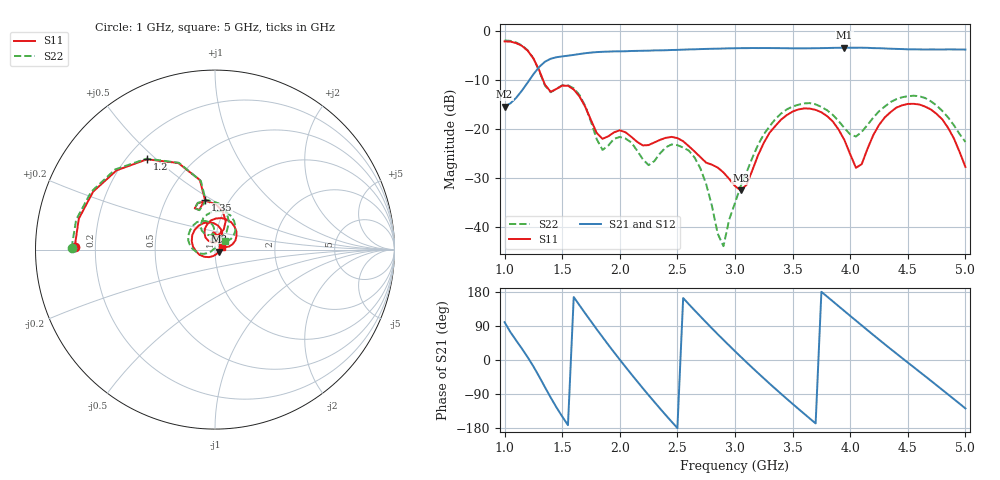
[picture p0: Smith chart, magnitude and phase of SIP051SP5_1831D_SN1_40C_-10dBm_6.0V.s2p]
# GHz  S  dB  R  50
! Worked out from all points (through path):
!   81 points, 1 GHz to 5 GHz, reference 50 ohm
!   highest |S21| = -3.42 dB at 3.95 GHz (marker M1); lowest = -15.5 dB at 1 GHz (marker M2)
!   lowest |S11| = -32.6 dB at 3.05 GHz (marker M3), VSWR 1.05, Z = 52.1 - j1.21 ohm
!   |S11| at or under -10 dB: 1.333 GHz to end of sweep
!   |S22| runs from -44.0 to -1.9 dB; largest |S21 - S12| = 0.0038
!   S11 on the Smith chart (normalised r, x): 1 GHz: 0.12, +0.01; 1.2 GHz: 0.28, +0.47; 1.35 GHz: 0.77, +0.46; 5 GHz: 1.08, +0.04
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1  -2.14 179.0  -15.46 99.7  -15.47 99.5  -1.94 179.5
1.2  -4.02 127.0  -10.56 7.5  -10.53 7.5  -3.96 126.9
1.35  -10.98 101.4  -6.30 -71.6  -6.30 -71.7  -11.16 100.6
1.55  -11.22 100.2  -5.05 -171.9  -5.05 -171.9  -11.10 98.7
1.7  -15.51 69.3  -4.55 123.0  -4.57 123.0  -15.34 62.8
1.85  -22.05 87.4  -4.26 60.5  -4.27 60.4  -24.33 82.5
2  -20.31 94.9  -4.17 0.9  -4.17 0.8  -21.68 94.3
2.2  -23.40 91.6  -4.05 -74.6  -4.05 -74.5  -26.25 82.7
2.35  -22.26 96.7  -3.97 -128.3  -3.96 -128.3  -25.01 111.6
2.5  -21.91 79.3  -3.87 -179.7  -3.87 -179.7  -23.36 89.6
2.7  -25.81 61.2  -3.71 115.0  -3.72 114.9  -28.12 54.9
2.9  -28.93 42.8  -3.59 53.0  -3.58 52.9  -44.00 140.7
3  -31.71 6.2  -3.54 23.1  -3.53 23.3  -35.16 -159.8
3.05  -32.61 -29.7  -3.52 8.5  -3.52 8.4  -31.68 -154.0
3.4  -18.13 172.0  -3.52 -89.3  -3.52 -89.3  -16.88 169.1
3.7  -16.14 102.8  -3.53 -167.3  -3.54 -167.3  -15.02 115.6
3.95  -22.32 62.3  -3.42 129.2  -3.44 129.2  -19.86 93.2
4.05  -27.97 85.3  -3.43 103.9  -3.43 104.0  -21.58 107.8
4.35  -16.61 107.0  -3.63 29.3  -3.64 29.4  -14.53 110.1
4.55  -14.90 69.1  -3.76 -18.6  -3.76 -18.7  -13.25 78.2
4.75  -16.96 32.4  -3.79 -66.7  -3.79 -66.7  -15.23 49.0
5  -27.80 25.0  -3.80 -127.8  -3.80 -127.4  -22.68 39.1
